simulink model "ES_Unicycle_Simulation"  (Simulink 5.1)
settings: Solver=ode45  StartTime=0.0  StopTime=tmax  FixedStep=deltaT  MaxStep=deltaT+ .001  MinStep=deltaT-.001  RelTol=1e-3
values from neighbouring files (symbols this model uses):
  a = 0.1    [ES_Unicycle_nc_values_tune_V.m]    (also in ES_Unicycle_nc_values_tune_V_moving.m = 0.04; ES_Unicycle_Values.m = 0.05; gradient2.m = 2*(df2 - df1); abs_perturbation.m = 0.01)
  cx = 20    [ES_Unicycle_Values.m]    (also in ES_Unicycle_Values_SI.m = 10; ES_PointMass_Values.m; ES_SimplifyPointMass_Values.m = 15; ES_Unstable_Values.m = 15)
  cy = 20    [ES_Unicycle_Values.m]    (also in ES_Unicycle_Values_SI.m = 10; ES_PointMass_Values.m; ES_SimplifyPointMass_Values.m = 15; ES_Unstable_Values.m = 15)
  ICx = 2 - r    (= 1.8)    [ES_Unicycle_nc_values_tune_V.m]    (also in ES_Unicycle_nc_values_tune_V_moving.m = 1.5; ES_Unicycle_Values.m = 2; ES_Unicycle_Values_SI.m = 1; ES_PointMass_Values.m = 1)
  ICy = 2    [ES_Unicycle_nc_values_tune_V.m]    (also in ES_Unicycle_nc_values_tune_V_moving.m; ES_Unicycle_Values.m = 1; ES_Unicycle_Values_SI.m = 1; ES_PointMass_Values.m = 1)
  px = 1    [ES_Unicycle_Values.m]    (also in doublepointmass.m = -6)
  py = 1/2    (= 0.5)    [ES_Unicycle_Values.m]    (also in doublepointmass.m = -6)
  W = 0.03    [ES_Unicycle_nc_values_tune_V_moving.m]    (also in ES_Unicycle_Values.m = 20; ltiesc_steep_derivatives_trackr_dac.m = 20)
libraries: simulink x2

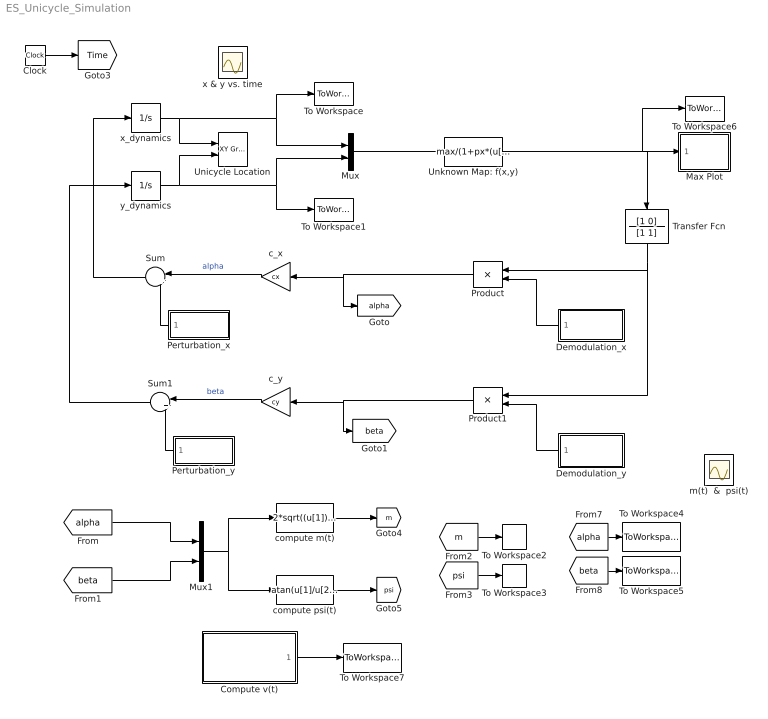
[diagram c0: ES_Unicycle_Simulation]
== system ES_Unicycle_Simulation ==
  Clock : Clock
  Compute v(t) : Subsystem
  Demodulation_x : Subsystem  Orientation=left
  Demodulation_y : Subsystem  Orientation=left
  Max Plot : Subsystem
  Mux : Mux  Inputs=2
  Mux1 : Mux  Inputs=2
  Perturbation_x : Subsystem  Orientation=left
  Perturbation_y : Subsystem  Orientation=left
  Product : Product  Orientation=left
  Product1 : Product  Orientation=left
  Sum : Sum  Orientation=left  Inputs=|++
  Sum1 : Sum  Orientation=left  Inputs=|++
  To Workspace : ToWorkspace  VariableName=X  SampleTime=-1  SaveFormat=Array
  To Workspace1 : ToWorkspace  VariableName=Y  SampleTime=-1  SaveFormat=Array
  To Workspace2 : ToWorkspace  VariableName=m  SampleTime=-1  SaveFormat=Array
  To Workspace3 : ToWorkspace  VariableName=psi  SampleTime=-1  SaveFormat=Array
  To Workspace4 : ToWorkspace  VariableName=alpha  SampleTime=-1  SaveFormat=Array
  To Workspace5 : ToWorkspace  VariableName=beta  SampleTime=-1  SaveFormat=Array
  To Workspace6 : ToWorkspace  VariableName=MAX  SampleTime=-1  SaveFormat=Array
  To Workspace7 : ToWorkspace  VariableName=v  SampleTime=-1  SaveFormat=Array
  Transfer Fcn : TransferFcn  Orientation=down  Numerator=[1 0]  Denominator=[1 1]
  Unicycle Location : simulink/Sinks/XY Graph  xmin=-abs(ICx) - 2  xmax=abs(ICx) + 1  ymin=-abs(ICy) - 2  ymax=abs(ICy) + 1  st=-1
  Unknown Map: f(x,y) : Fcn  Expr=max/(1+px*(u[1])^2+py*(u[2])^2)
  c_x : Gain  Orientation=left  Gain=cx
  c_y : Gain  Orientation=left  Gain=cy
  compute m(t) : Fcn  Expr=2*sqrt((u[1])^2+(u[2])^2)
  compute psi(t) : Fcn  Expr=atan(u[1]/u[2])
  m(t)  &  psi(t) : Scope  NumInputPorts=2
  x & y vs. time : Scope  NumInputPorts=2
  x_dynamics : Integrator  InitialCondition=ICx
  y_dynamics : Integrator  InitialCondition=ICy
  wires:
  Unknown Map: f(x,y)/1 -> Max Plot/1(ES Value), To Workspace6/1, Transfer Fcn/1
  Sum/1 -> x_dynamics/1
  Sum1/1 -> y_dynamics/1
  c_x/1 -> Sum/1  "alpha"
  c_y/1 -> Sum1/1  "beta"
  Perturbation_x/1(Perturbation) -> Sum/2
  Perturbation_y/1(Perturbation) -> Sum1/2
  Mux/1 -> Unknown Map: f(x,y)/1
  x_dynamics/1 -> Mux/1, To Workspace/1, Unicycle Location/1
  y_dynamics/1 -> Mux/2, To Workspace1/1, Unicycle Location/2
  [alpha] -> Mux1/1
  Mux1/1 -> compute psi(t)/1, compute m(t)/1
  compute m(t)/1 -> [m]
  compute psi(t)/1 -> [psi]
  Product/1 -> c_x/1, [alpha]
  Product1/1 -> c_y/1, [beta]
  Clock/1 -> [Time]
  [beta] -> Mux1/2
  [alpha] -> To Workspace4/1
  [beta] -> To Workspace5/1
  Demodulation_y/1(Demodulation) -> Product1/2
  Demodulation_x/1(Demodulation) -> Product/2
  [m] -> To Workspace2/1
  [psi] -> To Workspace3/1
  Transfer Fcn/1 -> Product/1, Product1/1
  Compute v(t)/1(Input to Unicycle) -> To Workspace7/1

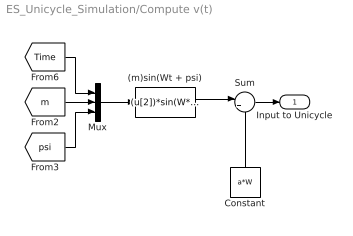
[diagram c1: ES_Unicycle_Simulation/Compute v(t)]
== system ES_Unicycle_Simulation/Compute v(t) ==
  (m)sin(Wt + psi) : Fcn  Expr=(u[2])*sin(W*u[1] + u[3])
  Constant : Constant  Orientation=up  Value=a*W
  Mux : Mux  Inputs=3
  Sum : Sum  Inputs=|++
  Input to Unicycle : Outport
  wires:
  Constant/1 -> Sum/2
  [Time] -> Mux/1
  Mux/1 -> (m)sin(Wt + psi)/1
  [psi] -> Mux/3
  [m] -> Mux/2
  (m)sin(Wt + psi)/1 -> Sum/1
  Sum/1 -> Input to Unicycle/1

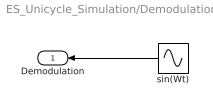
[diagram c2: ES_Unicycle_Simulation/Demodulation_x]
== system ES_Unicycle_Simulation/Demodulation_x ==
  sin(Wt) : Sin  Orientation=left  Frequency=W  SampleTime=0
  Demodulation : Outport  Orientation=left
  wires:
  sin(Wt)/1 -> Demodulation/1

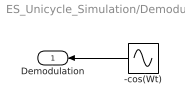
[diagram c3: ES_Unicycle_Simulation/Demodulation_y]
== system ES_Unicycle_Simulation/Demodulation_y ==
  -cos(Wt) : Sin  Orientation=left  Amplitude=-1  Frequency=W  Phase=pi/2  SampleTime=0
  Demodulation : Outport  Orientation=left
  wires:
  -cos(Wt)/1 -> Demodulation/1

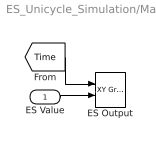
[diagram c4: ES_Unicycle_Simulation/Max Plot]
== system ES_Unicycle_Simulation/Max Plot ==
  ES Value : Inport
  ES Output : simulink/Sinks/XY Graph  xmin=0  xmax=tmax  ymin=max - 3  ymax="max  + 2"  st=-1
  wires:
  [Time] -> ES Output/1
  ES Value/1 -> ES Output/2

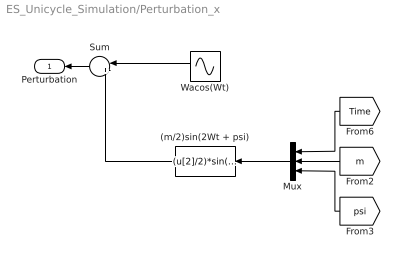
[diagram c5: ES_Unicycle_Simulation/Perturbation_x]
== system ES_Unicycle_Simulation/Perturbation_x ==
  (m/2)sin(2Wt + psi) : Fcn  Orientation=left  Expr=(u[2]/2)*sin(2*W*u[1] + u[3])
  Mux : Mux  Orientation=left  Inputs=3
  Sum : Sum  Orientation=left  Inputs=|++
  Wacos(Wt) : Sin  Orientation=left  Amplitude=W*a  Frequency=W  Phase=pi/2  SampleTime=0
  Perturbation : Outport  Orientation=left
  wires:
  (m/2)sin(2Wt + psi)/1 -> Sum/2
  Wacos(Wt)/1 -> Sum/1
  Sum/1 -> Perturbation/1
  [Time] -> Mux/1
  Mux/1 -> (m/2)sin(2Wt + psi)/1
  [psi] -> Mux/3
  [m] -> Mux/2

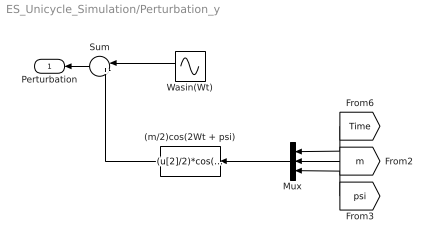
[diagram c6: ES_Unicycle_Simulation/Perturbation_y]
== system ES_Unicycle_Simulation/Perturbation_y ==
  (m/2)cos(2Wt + psi) : Fcn  Orientation=left  Expr=(u[2]/2)*cos(2*W*u[1] + u[3])
  Mux : Mux  Orientation=left  Inputs=3
  Sum : Sum  Orientation=left  Inputs=|+-
  Wasin(Wt) : Sin  Orientation=left  Amplitude=W*a  Frequency=W  SampleTime=0
  Perturbation : Outport  Orientation=left
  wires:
  (m/2)cos(2Wt + psi)/1 -> Sum/2
  Wasin(Wt)/1 -> Sum/1
  Sum/1 -> Perturbation/1
  [Time] -> Mux/1
  Mux/1 -> (m/2)cos(2Wt + psi)/1
  [psi] -> Mux/3
  [m] -> Mux/2
